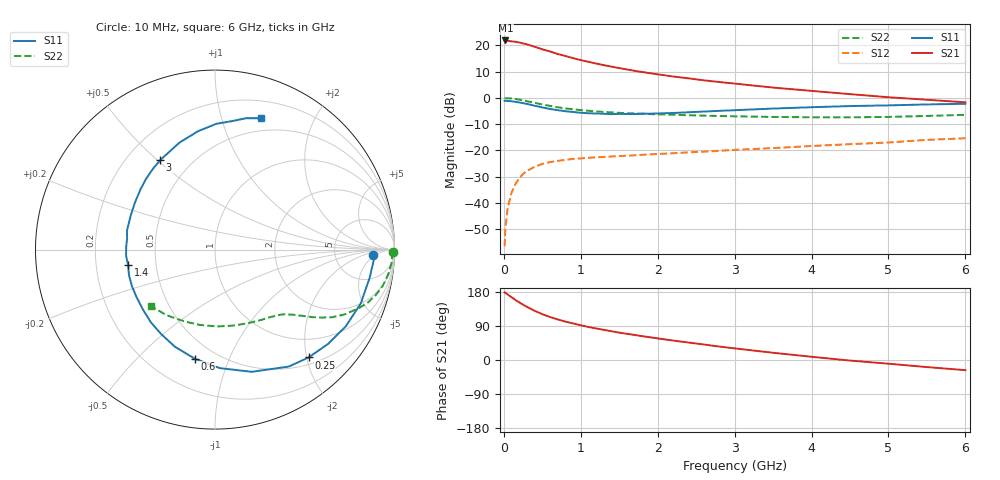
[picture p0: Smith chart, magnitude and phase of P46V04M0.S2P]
! SIEMENS Small Signal Semiconductors
! BFP182
! Si NPN RF Bipolar Junction Transistor in SOT143
! VCE = 6 V  IC = 4 mA
! Common Emitter S-Parameters:  March  1996
# GHz  S  MA  R  50
!  f  S11  S21  S12  S22
! GHz  MAG  ANG  MAG  ANG  MAG  ANG  MAG  ANG
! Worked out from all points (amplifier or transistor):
!   36 points, 10 MHz to 6 GHz, reference 50 ohm
!   highest |S21| = 21.9 dB at 20 MHz (marker M1)
!   |S21| within 3 dB of that: start of sweep to 461.5 MHz
!   unconditionally stable (mu >= 1): 1.81 GHz to 5.693 GHz
!   at 250 MHz: K = 0.18, MSG = 24.9 dB, |S12| = -29.0 dB
!   at 1.4 GHz: K = 0.85, MSG = 17.1 dB, |S12| = -22.3 dB
!   at 6 GHz: K = 0.96, MSG = 6.8 dB, |S12| = -15.4 dB
!   S11 on the Smith chart (normalised r, x): 10 MHz: 15, -4; 250 MHz: 0.62, -2.04; 600 MHz: 0.38, -0.75; 1.4 GHz: 0.34, -0.08; 3 GHz: 0.34, +0.51; 6 GHz: 0.37, +1.34
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0.01  0.8823 -2.0  12.27 178.6  0.0015 81.7  0.9924 -0.8
0.02  0.8857 -4.1  12.46 177.4  0.0033 90.7  0.9876 -1.6
0.05  0.8759 -10.3  12.25 172.8  0.008 88.5  0.987 -4.2
0.15  0.8445 -30.5  11.78 158.7  0.0228 73.6  0.9556 -12.3
0.2  0.8206 -39.7  11.4 152.1  0.0294 69.0  0.9306 -15.8
0.25  0.7959 -49.0  10.94 145.8  0.0356 64.0  0.9015 -19.1
0.3  0.7703 -57.8  10.53 140.4  0.0408 60.3  0.8684 -21.9
0.4  0.7108 -73.3  9.449 129.8  0.0487 53.1  0.8074 -26.6
0.5  0.6609 -87.7  8.451 121.0  0.0554 47.2  0.7536 -30.0
0.6  0.6178 -100.6  7.687 113.5  0.0601 43.1  0.7047 -32.5
0.7  0.5858 -112.3  6.886 107.1  0.0633 39.7  0.6653 -34.5
0.8  0.5586 -122.3  6.305 101.3  0.066 37.2  0.6326 -36.1
1  0.522 -140.4  5.255 91.6  0.0704 33.6  0.5872 -38.6
1.1  0.5109 -148.9  4.886 87.1  0.0725 32.5  0.5693 -39.6
1.4  0.4917 -170.0  3.948 75.9  0.0767 30.4  0.5304 -42.8
1.8  0.5022 167.8  3.121 62.8  0.0826 29.0  0.4999 -47.5
2.2  0.5173 149.5  2.565 51.3  0.0883 28.6  0.4783 -53.2
3  0.5846 121.5  1.879 30.7  0.1024 27.4  0.4471 -67.0
3.5  0.628 108.4  1.577 19.1  0.1109 26.0  0.4348 -77.1
4.5  0.701 89.4  1.183 -1.5  0.1316 22.7  0.4279 -101.0
5.5  0.7526 76.6  0.924 -18.7  0.1589 18.7  0.4544 -126.5
6  0.7749 70.8  0.825 -26.8  0.1707 14.8  0.4767 -138.9
